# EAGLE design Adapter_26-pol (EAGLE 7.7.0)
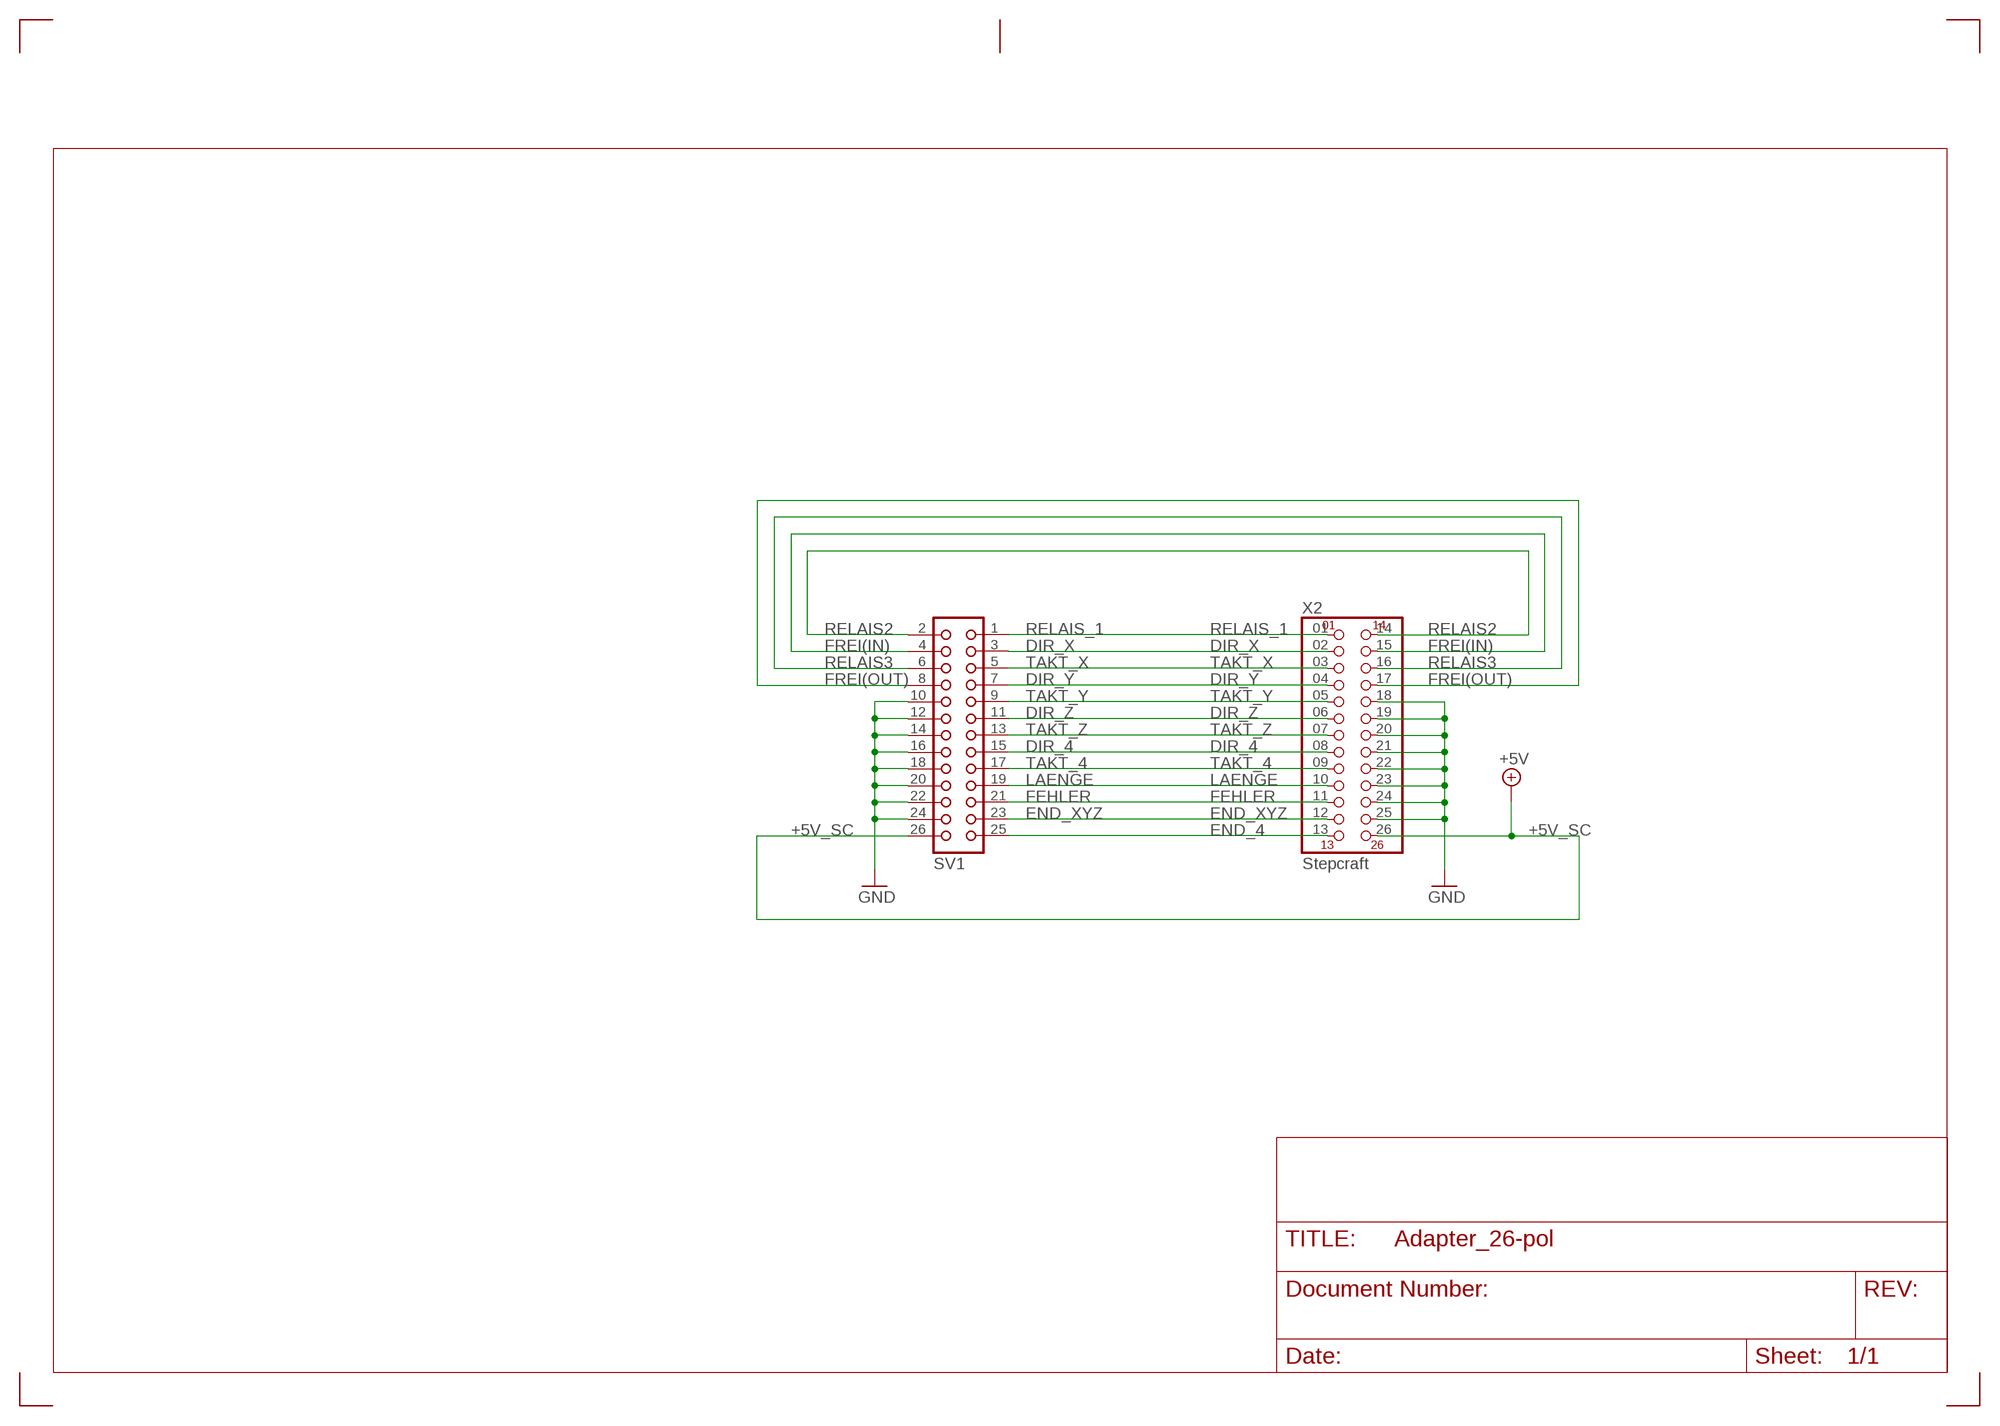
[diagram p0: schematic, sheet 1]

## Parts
SV1  CON26L  [CON26L]
X2  Stepcraft  PINHD-2X13_STEPCRAFT  [2X13_90_STEPCRAFT]

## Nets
+5V_SC: SV1.26 X2.26 ; supply symbol labelled +5V
DIR_4: SV1.15 X2.08
DIR_X: SV1.3 X2.02
DIR_Y: SV1.7 X2.04
DIR_Z: SV1.11 X2.06
END_4: SV1.25 X2.13
END_XYZ: SV1.23 X2.12
FEHLER: SV1.21 X2.11
FREI(IN): SV1.4 X2.15
FREI(OUT): SV1.8 X2.17
GND: SV1.10 SV1.12 SV1.14 SV1.16 SV1.18 SV1.20 SV1.22 SV1.24 X2.18 X2.19 X2.20 X2.21 X2.22 X2.23 X2.24 X2.25
LAENGE: SV1.19 X2.10
RELAIS2: SV1.2 X2.14
RELAIS3: SV1.6 X2.16
RELAIS_1: SV1.1 X2.01
TAKT_4: SV1.17 X2.09
TAKT_X: SV1.5 X2.03
TAKT_Y: SV1.9 X2.05
TAKT_Z: SV1.13 X2.07

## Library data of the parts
SV1 = con-harting:CON26L: CONNECTOR; OC_FARNELL: unknown; OC_NEWARK: unknown
X2 = con-pinhead:PINHD-2X13_STEPCRAFT

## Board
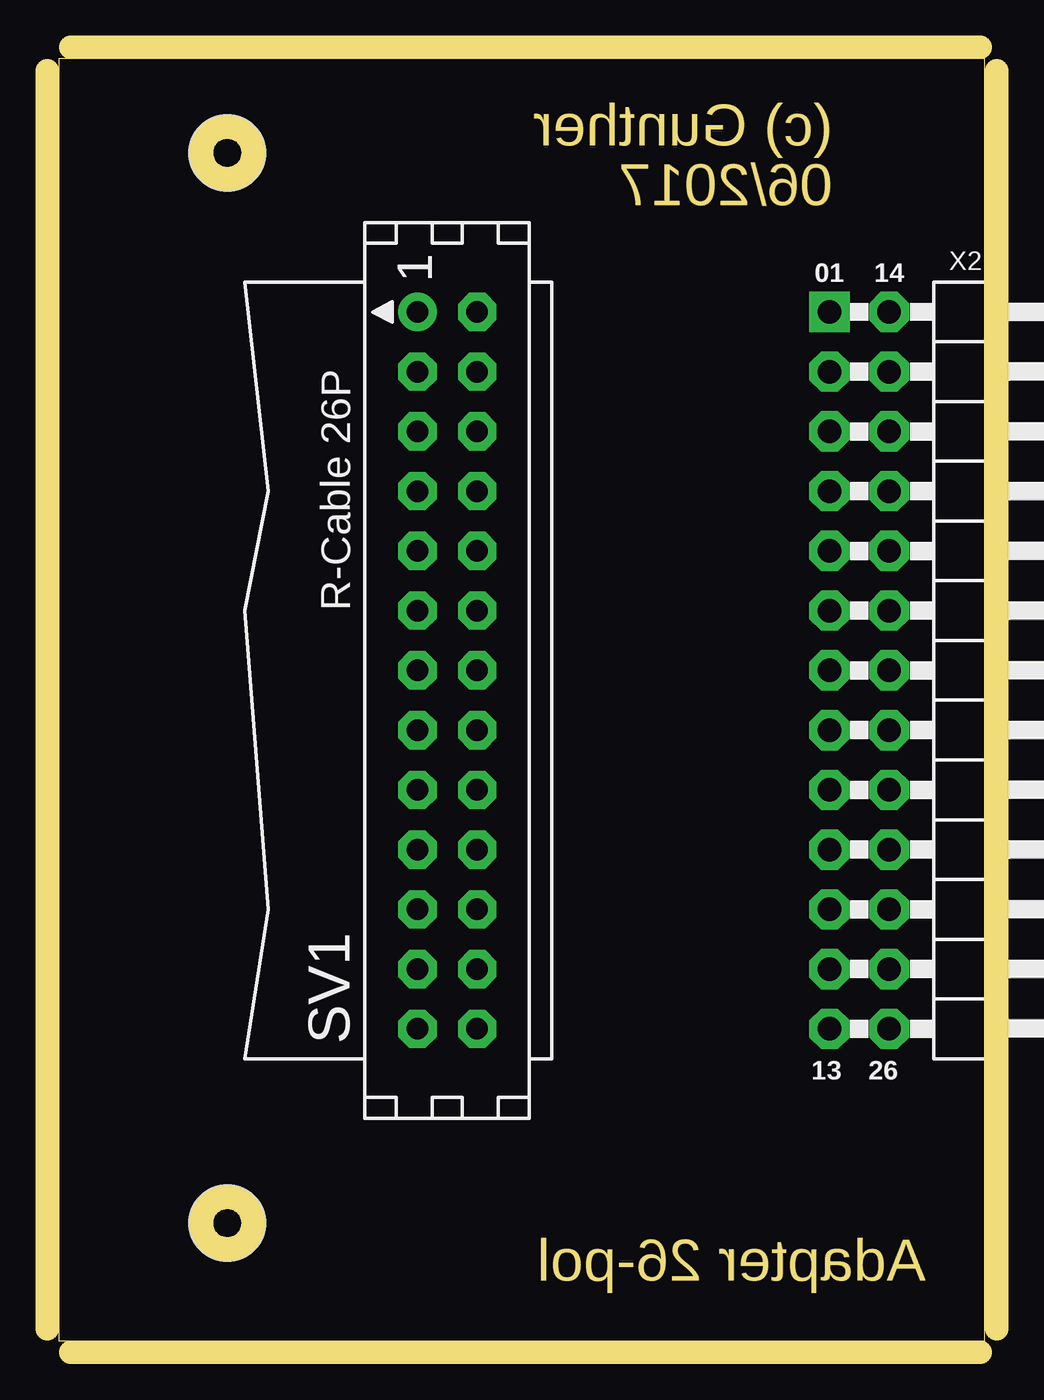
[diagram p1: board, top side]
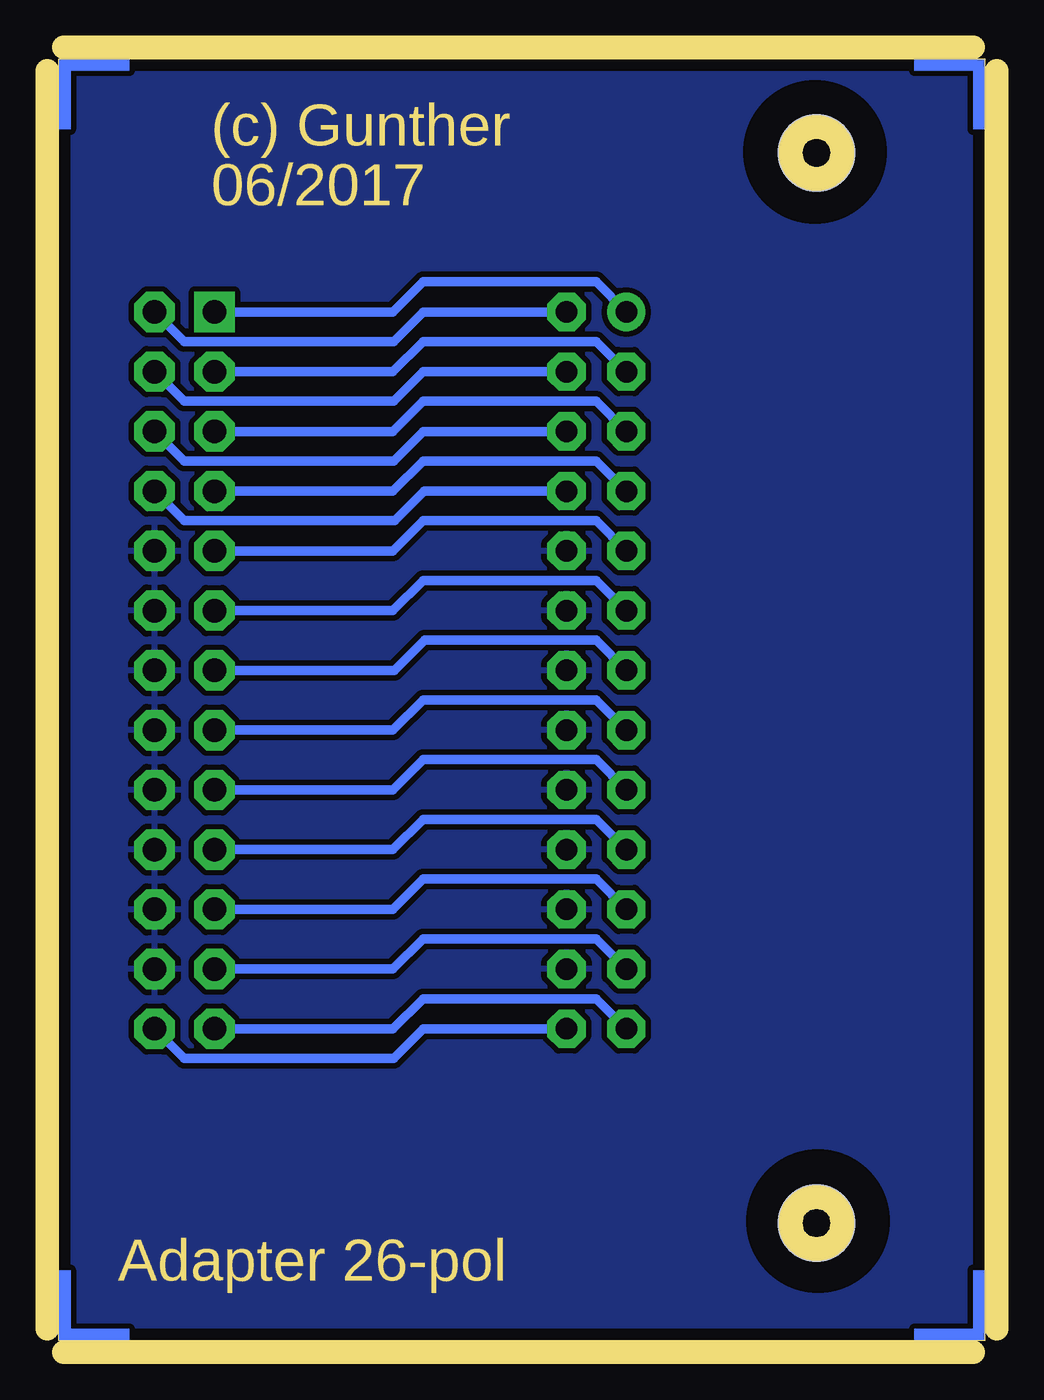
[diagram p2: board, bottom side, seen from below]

Size 39.36 x 54.5 mm. Coordinates in mm from the lower left corner, seen from the top.
Outline: 0,0 39.36,0 39.36,54.5 0,54.5 0,0
Copper layers (1*16): Top 0.035mm / dielectric 1.5mm / Bottom 0.035mm
Design rules "LP_fraesen *": minimum track width 12mil, minimum drill 23mil, track to track 8mil, track to pad 8mil, pad to pad 8mil, via to via 8mil, smd to smd 0mil, copper to edge 20mil, drill to drill 8mil, minimum pad ring 14mil, minimum via ring 15mil, stop-mask expansion 4mil, vias tented up to drill 0mil, thermal gap 10mil
Holes 3.2 mm at 7.16,50.5 7.16,5
bRestrict: area 4.6,47.9 to 9.9,53.2; area 4.4,2.4 to 9.8,7.7
Milling: 10 lines

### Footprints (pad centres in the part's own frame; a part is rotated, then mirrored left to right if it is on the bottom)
CON26L = drill 0.914: 1 15.24,1.27 | drill 0.914 octagon: 2 15.24,-1.27; 3 12.7,1.27; 4 12.7,-1.27; 5 10.16,1.27; 6 10.16,-1.27; 7 7.62,1.27; 8 7.62,-1.27; 9 5.08,1.27; 10 5.08,-1.27; 11 2.54,1.27; 12 2.54,-1.27; 13 0,1.27; 14 0,-1.27; 15 -2.54,1.27; 16 -2.54,-1.27; 17 -5.08,1.27; 18 -5.08,-1.27; 19 -7.62,1.27; 20 -7.62,-1.27; 21 -10.16,1.27; 22 -10.16,-1.27; 23 -12.7,1.27; 24 -12.7,-1.27; 25 -15.24,1.27; 26 -15.24,-1.27
2X13_90_STEPCRAFT = drill 1 square: 01 -15.24,-1.27 | drill 1 octagon: 02 -12.7,-1.27; 03 -10.16,-1.27; 04 -7.62,-1.27; 05 -5.08,-1.27; 06 -2.54,-1.27; 07 0,-1.27; 08 2.54,-1.27; 09 5.08,-1.27; 10 7.62,-1.27; 11 10.16,-1.27; 12 12.7,-1.27; 13 15.24,-1.27; 14 -15.24,1.27; 15 -12.7,1.27; 16 -10.16,1.27; 17 -7.62,1.27; 18 -5.08,1.27; 19 -2.54,1.27; 20 0,1.27; 21 2.54,1.27; 22 5.08,1.27; 23 7.62,1.27; 24 10.16,1.27; 25 12.7,1.27; 26 15.24,1.27

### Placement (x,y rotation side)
SV1  16.51,28.5 90 top
X2  34.02,28.5 270 top

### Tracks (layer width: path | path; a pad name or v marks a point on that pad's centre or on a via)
+5V_SC
  Bottom 0.406: X2.26 34.03,12 25.13,12 23.88,13.26 SV1.26
DIR_4
  Bottom 0.406: SV1.15 16.52,27.24 23.88,27.24 25.16,25.96 X2.08
DIR_X
  Bottom 0.406: SV1.3 16.52,42.48 23.88,42.48 25.16,41.2 X2.02
DIR_Y
  Bottom 0.406: SV1.7 16.52,37.4 23.88,37.4 25.16,36.12 X2.04
DIR_Z
  Bottom 0.406: SV1.11 16.52,32.32 23.88,32.32 25.16,31.04 X2.06
END_4
  Bottom 0.406: SV1.25 16.52,14.54 23.88,14.54 25.16,13.26 X2.13
END_XYZ
  Bottom 0.406: SV1.23 16.52,17.08 23.88,17.08 25.16,15.8 X2.12
FEHLER
  Bottom 0.406: SV1.21 16.52,19.62 23.88,19.62 25.16,18.34 X2.11
FREI(IN)
  Bottom 0.406: X2.15 34.03,39.94 25.13,39.94 23.88,41.2 SV1.4
FREI(OUT)
  Bottom 0.406: X2.17 34.03,34.86 25.08,34.86 23.82,36.12 SV1.8
GND
  pour Bottom (isolate 0.229, rank 3): 0,0 39.67,0 39.67,54.48 0,54.48
LAENGE
  Bottom 0.406: SV1.19 16.52,22.16 23.88,22.16 25.16,20.88 X2.10
RELAIS2
  Bottom 0.406: X2.14 34.03,42.48 25.13,42.48 23.88,43.74 SV1.2
RELAIS3
  Bottom 0.406: X2.16 34.03,37.4 25.13,37.4 23.88,38.66 SV1.6
RELAIS_1
  Bottom 0.406: SV1.1 16.52,45.02 23.88,45.02 25.16,43.74 X2.01
TAKT_4
  Bottom 0.406: SV1.17 16.52,24.7 23.88,24.7 25.16,23.42 X2.09
TAKT_X
  Bottom 0.406: SV1.5 16.52,39.94 23.88,39.94 25.16,38.66 X2.03
TAKT_Y
  Bottom 0.406: SV1.9 16.52,34.86 23.88,34.86 25.16,33.58 X2.05
TAKT_Z
  Bottom 0.406: SV1.13 16.52,29.78 23.81,29.78 25.09,28.5 X2.07
(copper drawn outside any net)
  shapes: Bottom area x8

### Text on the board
Milling: (c) Gunther | 06/2017 | Adapter 26-pol
Reference: 10 | 20 | 30 | 40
